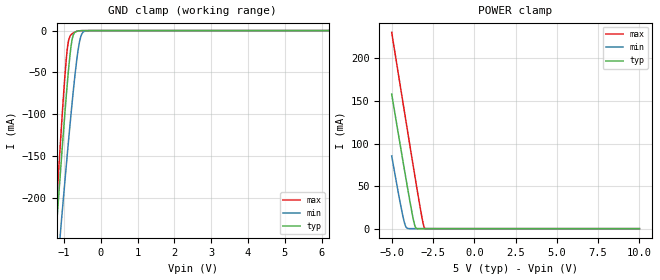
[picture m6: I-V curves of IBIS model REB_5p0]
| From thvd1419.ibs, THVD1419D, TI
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|   REB_5p0 Model
[Model]   REB_5p0
Model_type   Input
Vinl = 0.8
Vinh = 2
|   typ   min   max
C_comp   3.481pF   2.962pF   4.015pF
| Where Nom  PVT is Nominal Process, 5.0V, 25C
|   Fast PVT is Strong Process,  5.5V, -40C
|   Slow PVT is Weak Process,   4.5V, 150C
[Voltage Range]   5   4.5   5.5
|Junction Temperature
[Temperature Range]   25   150   -40
[Power Clamp Reference]   5   4.5   5.5
[GND Clamp Reference]   0   0   0
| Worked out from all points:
|   GND clamp passes 1 mA (typ) near -0.66 V on its own axis
|   POWER clamp passes 1 mA (typ) near -3.54 V on its own axis
[GND Clamp]
|   Voltage   I(typ)   I(min)   I(max)
-5V       -2.704A    -2.364A    -3.147A
-1.235V   -255.2mA   -314.4mA   -234.6mA
-1.145V   -200mA     -267.7mA   -169.5mA
-1.07V    -154.9mA   -229.3mA   -117.1mA
-965mV    -94.34mA   -176.3mA   -50.1mA
-905mV    -62.15mA   -146.8mA   -21.15mA
-860mV    -40.29mA   -125.1mA   -9.613mA
-785mV    -12.81mA   -90.15mA   -4.089mA
-650mV    -852.6uA   -34.76mA   -894.9uA
-545mV    -147.7uA   -7.74mA    -141.3uA
-410mV    -13.32uA   -354.9uA   -9.554uA
10V       0A         0A         0A
[POWER Clamp]
|   Voltage   I(typ)   I(min)   I(max)
-5V       157.9mA    85.38mA    230.5mA
-4.46V    95.51mA    27.84mA    165.2mA
-4.265V   73.22mA    9.808mA    141.7mA
-4.16V    61.32mA    3.054mA    129.1mA
-4.055V   49.53mA    438.7uA    116.4mA
-3.77V    18.7mA     225.5nA    82.38mA
-3.59V    3.072mA    7.023nA    61.06mA
-3.485V   191.4uA    375pA      48.74mA
-3.14V    0A         0A         10.25mA
-3.05V    0A         0A         2.66mA
-2.99V    0A         0A         420.2uA
10V       0A         0A         0A
